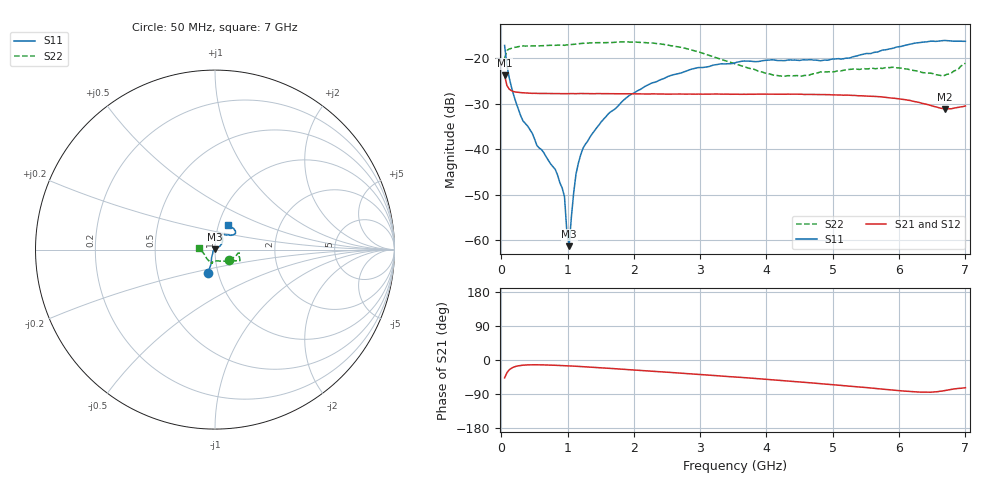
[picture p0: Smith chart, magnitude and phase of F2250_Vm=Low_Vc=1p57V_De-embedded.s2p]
! Integrated Device Technology
! Corporate Headquarters
! 6024 Silver Creek Valley Road
! San Jose, CA 95138  USA
! Phone:  1-408-284-8200
! Toll Free:  1-800-223-1366
! Webpage:  http://www.idt.com/
! Timing and RF Division
! 515 Groton Road, Suite 102
! Westford, MA 01886-6024
! Device:  F2250
! Description: Voltage Variable RF Attenuator
! Frequency:  50.0 -  6000.00 MHz
! Package:  3x3 mm Thin QFN Plastic Package: 16 pin
! Ports:  2 RF, 3 DC
!  Pin  1  = GND
!  Pin  2  = NC
!  Pin  3  = RF1  = Port 1
!  Pin  4  = NC
!  Pin  5  = GND
!  Pin  6  = GND
!  Pin  7  = GND
!  Pin  8  = GND
!  Pin  9  = NC
!  Pin 10  = RF2  = Port 2
!  Pin 11  = NC
!  Pin 12  = GND
!  Pin 13  = GND
!  Pin 14  = VCNTRL
!  Pin 15  = VDD
!  Pin 16  = VMODE
! Vcntrl:  1.570 Volts
! Vmode:  +0.000 Volts
! Vdd:  +3.30  Volts
! Current:  1.189 mA
! Data:  The device was measured on a the F2250 evaluation board which has
!  individual transmission lines to the RF pins.  Data was collected
!  using a calibrated network analyzer.  The evaluation board was
!  de-embedded using a TRL calibration technique.
!  The reference plane is the edge of the package pin.
! Misc:  SN 10
!  Action Tracker AT0258
! Date Measured:  2014-11-26
! Date:  2015-10-15  MJV
! Note:
!  Integrated Device Technology supplies this data as a sample of measured
!  data at the package pin for this product.  Your particular data for this
!  product may vary.
!  Data was taken at 25 degrees C.
!  Integrated Device Technology reserves the right to change this data at anytime.
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# GHz S dB R 50
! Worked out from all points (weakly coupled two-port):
!   201 points, 50 MHz to 7 GHz, reference 50 ohm
!   highest |S21| = -23.78 dB at 50 MHz (marker M1); lowest = -31.1 dB at 6.687 GHz (marker M2)
!   lowest |S11| = -61.3 dB at 1.023 GHz (marker M3), VSWR 1.00, Z = 50 + j0.0844 ohm
!   |S11| at or under -10 dB: start of sweep to end of sweep
!   |S22| runs from -23.9 to -16.4 dB; largest |S21 - S12| = 0.0002
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0.05  -17.18 -107.1  -23.78 -47.1  -23.78 -47.1  -20.01 -36.9
0.1195  -24.28 -109.0  -26.78 -26.0  -26.80 -26.0  -17.96 -11.4
0.29325  -32.67 -121.4  -27.55 -14.3  -27.56 -14.3  -17.33 -8.6
0.5365  -39.15 -146.6  -27.72 -12.6  -27.73 -12.6  -17.29 -9.8
0.8145  -44.45 176.9  -27.78 -13.9  -27.77 -13.9  -17.14 -14.0
0.91875  -48.54 155.1  -27.78 -14.7  -27.80 -14.7  -17.08 -15.8
0.9535  -50.46 177.7  -27.78 -15.0  -27.81 -15.0  -17.15 -16.0
0.98825  -58.03 159.8  -27.78 -15.3  -27.80 -15.3  -17.06 -16.3
1.023  -61.32 79.2  -27.77 -15.6  -27.79 -15.5  -17.00 -16.4
1.0925  -49.51 36.3  -27.77 -16.2  -27.80 -16.2  -16.93 -17.3
1.12725  -45.43 33.4  -27.78 -16.5  -27.78 -16.5  -16.86 -17.9
1.2315  -39.81 29.3  -27.75 -17.6  -27.78 -17.6  -16.71 -19.4
1.5095  -33.95 32.6  -27.78 -20.7  -27.78 -20.7  -16.57 -21.3
1.82225  -29.50 35.0  -27.80 -24.3  -27.81 -24.3  -16.40 -23.5
2.37825  -24.86 44.6  -27.85 -30.8  -27.85 -30.8  -16.79 -26.2
2.93425  -22.15 58.1  -27.89 -37.4  -27.88 -37.5  -18.44 -30.9
3.525  -20.99 71.2  -27.90 -44.8  -27.90 -44.9  -21.20 -47.7
4.11575  -20.36 78.8  -27.92 -52.5  -27.92 -52.5  -23.74 -73.4
4.7065  -20.39 71.6  -27.96 -60.8  -27.94 -60.8  -23.41 -97.8
5.85325  -17.94 39.7  -28.68 -78.5  -28.66 -78.6  -22.06 -105.7
6.68725  -16.08 48.3  -31.13 -80.7  -31.10 -80.7  -23.76 -156.3
7  -16.26 62.8  -30.48 -73.2  -30.48 -73.2  -21.09 174.7
